PROGRAM FeedTable
VAR
	(*配置插补通道FB*)
   	FB_BuildNciGroup            : CfgBuildExt3DGroup;   //配置NCI通道
	FB_CfgReconfigGroup         : CfgReconfigGroup;     //解散NCI通道
	FB_StartStopG               : ItpStartStopEx;       //启动停止
	FB_ItpResetGroup            : ItpResetEx2;          //复位NCI通道
	UI_ItpState                 : UDINT;                //插补通道状态返回值
	L_Override                  : LREAL  :=100;         //插补通道速比
	
	(*FeedTable相关变量、功能块定义*)
	TablePrep				    : FB_NciFeedTablePreparation; //准备填充Nci Table
	NciFeedTable                : FB_NciFeedTable;            //执行Nci Table
    Nci_Command                 : Nci_SingleEntry;            //Nci单次指令输入
	GeoLine                     : ST_NciGeoLine;              //直线插补
	GeoCirclePlane		        : ST_NciGeoCirclePlane;       //圆弧插补
	EndOfTable                  : ST_NciEndOfTables;          
	Nci_Table				    : ST_NciFeedGroupTable;       //指令顺序表
	TableDisplayIndex	        : UDINT := 1;				  //插补指令在Table中的索引号
	FB_RtrigPrep                : R_Trig;                     //上升沿
	B_TablePrep                 : BOOL;                       //指令填充
	step                        : INT; 
	
	(*NcPTP指令*)
	FB_Power                    : ARRAY[1..AxisNum] OF MC_Power; //使能功能块
	B_Enable                    : BOOL;
	
	(*队列*)
	FB_CommandTable             :FB_PushPopStack;                //实例化队列功能块
	CommandArray                : ARRAY[1..100] OF Nci_SingleEntry;  //指令列表
	ClearCommandArray           :Bool;                               //清空触发位
END_VAR

A_LineTable();//FeedTable Nci 表格

A_NciChannel();//配置插补通道

A_NcPTP();//使能所有轴

ACTION A_LineTable:
FB_RtrigPrep(CLK:=B_TablePrep , Q=> );//上升沿触发存储一条Nci指令
IF FB_RtrigPrep.Q THEN;
	    TablePrep.bResetTable:=FALSE;
        IF 	Nci_Command .iPlane>0 THEN	 (* Circle平面圆弧插补*)
			GeoCirclePlane.fEndPosX	:=	REAL_TO_LREAL(Nci_Command .fx);
			GeoCirclePlane.fEndPosY	:=	REAL_TO_LREAL(Nci_Command .fy);
			GeoCirclePlane.fCenterX	:=	REAL_TO_LREAL(Nci_Command .fCenterX);
			GeoCirclePlane.fCenterY	:=	REAL_TO_LREAL(Nci_Command .fCenterY);
			GeoCirclePlane.fVelo    :=	REAL_TO_LREAL(Nci_Command .SyncVelo);
			GeoCirclePlane.bAccurateStop :=TRUE;
			TableDisplayIndex		:=	TableDisplayIndex+1; 
			GeoLine.nDisplayIndex 	:= 	TableDisplayIndex;
			TablePrep(
		    nEntryType		:=	GeoCirclePlane.nEntryType,
		    pEntry			:=	ADR(GeoCirclePlane),
		    stFeedGroupTable:= Nci_Table,
		    nFilledRows=>,
		    bError=>,
		    nErrorId=> );
            FB_CommandTable(ArrayNciCommand:=CommandArray , PushCommand:=Nci_Command , 
                            PopCommand=> , busy=> );
		    FB_CommandTable.PushStack();
		ELSE		                    (* Line直线插补*)
            
			GeoLine.fEndPosX		  :=	REAL_TO_LREAL(Nci_Command .fX);
			GeoLine.fEndPosY		  :=	REAL_TO_LREAL(Nci_Command .fY);
			GeoLine.fEndPosZ		  :=	REAL_TO_LREAL(Nci_Command .fZ);
			GeoLine.fEndPosQ1		  :=	REAL_TO_LREAL(Nci_Command .fQ1);
			GeoLine.fEndPosQ2		  :=	REAL_TO_LREAL(Nci_Command .fQ2);

			GeoLine.fVelo			  :=	REAL_TO_LREAL(Nci_Command .SyncVelo);
			GeoLine.nDisplayIndex 	  := 	TableDisplayIndex;
            
            TableDisplayIndex		    :=	TableDisplayIndex+1;
		    TablePrep(
		    nEntryType:=GeoLine.nEntryType,
		    pEntry:= ADR(GeoLine), 
		    stFeedGroupTable:= Nci_Table,
		    nFilledRows=>,
		    bError=>,
		    nErrorId=> );
            FB_CommandTable(ArrayNciCommand:=CommandArray , PushCommand:=Nci_Command , 
                            PopCommand=> , busy=> );
		     FB_CommandTable.PushStack();
		END_IF
	END_IF

CASE step OF
	0:
      IF NciFeedTable.bFeedingDone THEN //指令填充完毕便可以复位指令表
         TablePrep(
	       nEntryType:= , 
	       pEntry:= , 
	       bResetTable:=TRUE , 
	       bResetAll:= , 
	       stFeedGroupTable:=Nci_Table , 
	       nFilledRows=> , 
	       bError=> , 
	       nErrorId=> );
	     TableDisplayIndex :=1;	
	     step:=10;
      END_IF
	  
	10: 
	  NciFeedTable.bExecute:=FALSE;
	  TablePrep.bResetTable:=FALSE;
	  step:=0;
END_CASE
	
IF ClearCommandArray THEN       //清空指令队列
   FB_CommandTable.ClearStack();
   TablePrep(
	  nEntryType:= , 
	  pEntry:= , 
	  bResetTable:=TRUE , 
	  bResetAll:= , 
	  stFeedGroupTable:=Nci_Table , 
	  nFilledRows=> , 
	  bError=> , 
	  nErrorId=> );
   TableDisplayIndex    :=	1;
END_IF

		
NciFeedTable(
	bExecute:= , 
	bReset:= , 
	bLogFeederEntries:=FALSE , 
	stFeedGroupTable:=Nci_Table  , 
	stNciToPlc:=NciToPlc , 
);
END_ACTION

ACTION A_NciChannel:
(*NCI通道状态，通常用作标志位,uiItpState返回值代表着当前插补通道的状态，其中几个重要的状态：
  1：ITP_STATE_IDLE     该状态未加载任何G代码程序或是刚执行完复位功能，插补通道处于空闲状态。若当前执行G代码停止也会进入该状态。
  2: ITP_STATE_READY    成功导入G代码程序，插补通道进入准备状态。当G代码程序被完整执行完，插补通道也会进入该状态
  5: ITP_STATE_RUNNING  正在运行G代码
 12: ITP_STATE_ABORTED  如果在G代码运行过程中出现报错，插补通道立即进入该模式，当前报错代码也会出现在通道状态中*)
UI_ItpState	:=	ItpGetStateInterpreter(NciToPlc);//使用FeedTable形式进行插补该值不会变化
(*设置NCI通道的override*)
ItpSetOverridePercent(fOverridePercent:=L_Override, sPlcToNci:=	PlcToNci);
(*获取ID*)
GroupID := ItpGetGroupId(sNciToPlc:=NciToPlc );
ChannelID:=ItpGetChannelId(sNciToPlc:=NciToPlc );


(*功能块定义*)
IF B_Enable THEN //使能后直接将PTP轴配置进插补通道
   FB_BuildNciGroup.bExecute:=TRUE;
END_IF
FB_BuildNciGroup(
	bExecute:= , 
	nGroupId:=GroupID , 
	nXAxisId:=Nci_Axis[1].NcToPlc.AxisId , 
	nYAxisId:=Nci_Axis[2].NcToPlc.AxisId , 
	nZAxisId:=Nci_Axis[3].NcToPlc.AxisId, 
	tTimeOut:=T#300MS ,  );
	
FB_CfgReconfigGroup(
	bExecute:= , 
	nGroupId:=GroupID , 
	tTimeOut:=T#300MS , 
 );
 
 FB_StartStopG(
	bStart:= , 
	bStop:= , 
	tTimeOut:=T#300MS , 
	sNciToPlc:=NciToPlc , 
);

FB_ItpResetGroup(
	bExecute:= , 
	tTimeOut:=T#300MS , 
	sNciToPlc:=NciToPlc , 
 );
END_ACTION

ACTION A_NcPTP:
//轮询读取轴的状态
FOR i := 1 TO AxisNum BY 1 DO
    Nci_Axis[i].ReadStatus();
END_FOR

// 使能所有轴
IF B_Enable THEN
	FOR i := 1 TO AxisNum DO//用For语句进行使能
		FB_Power[i](
			Axis:= Nci_Axis[i], 
			Enable:= TRUE, 
			Enable_Positive:= TRUE, 
			Enable_Negative:= TRUE, 
			Override:= 100);
	END_FOR
END_IF
END_ACTION

END_PROGRAM
